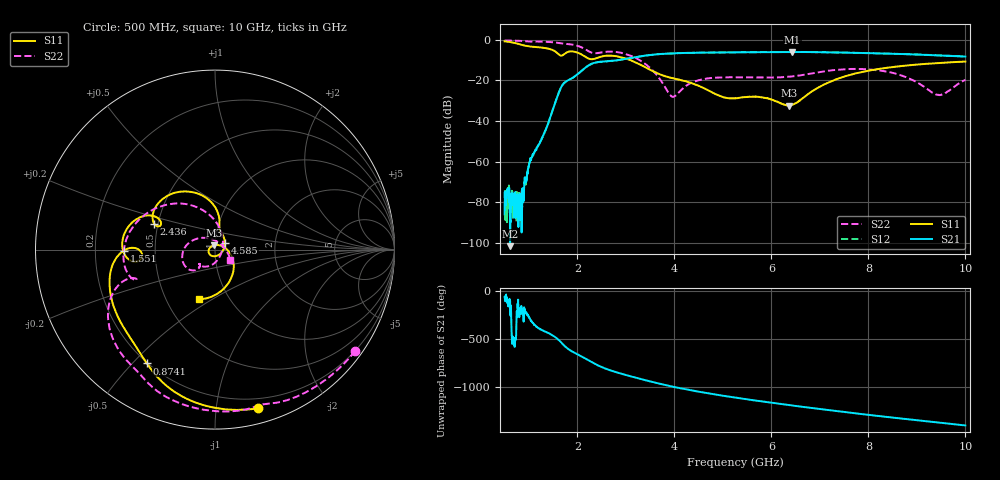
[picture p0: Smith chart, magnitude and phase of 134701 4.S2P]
!  2-Port S-parameters saved by WinCal
! VAR MeasName=S-Parameters (CALIBRATED_DATA) read from VNA (N5242A)
! VAR MeasDate=2013-7-3 16:21:27
! VAR NAME=134701 4
! VAR FILENAME=134701 4.S2P
! VAR DATE=2013-7-3 16:21:27
! VAR PHYS_PORTS=1,2
# Hz S MA R 50
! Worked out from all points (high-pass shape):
!   1601 points, 500 MHz to 10 GHz, reference 50 ohm
!   highest |S21| = -5.99 dB at 6.432 GHz (marker M1); lowest = -101.7 dB at 612.8 MHz (marker M2)
!   |S21| within 3 dB of the highest: 3.093 GHz to end of sweep
!   lowest |S11| = -32.5 dB at 6.372 GHz (marker M3), VSWR 1.05, Z = 49.4 + j2.27 ohm
!   |S11| at or under -10 dB: 3.09 GHz to end of sweep
!   |S22| runs from -28.1 to -0.3 dB; largest |S21 - S12| = 0.0033
!   S11 on the Smith chart (normalised r, x): 500 MHz: 0.12, -1.30; 874.1 MHz: 0.20, -0.55; 1.551 GHz: 0.33, -0.01; 2.436 GHz: 0.48, +0.16; 4.585 GHz: 1.11, +0.08; 10 GHz: 0.72, -0.44
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5e8  0.9167 -74.9  4.969e-05 -68.2  0.00013 -95.6  0.9631 -35.9
6.128125e8  0.8805 -90.3  8.261e-06 -99.5  0.0001217 127.1  0.9562 -43.9
8.146875e8  0.7737 -115.2  0.0001617 178.9  0.0001131 -93.5  0.9411 -58.3
8.740625e8  0.7392 -120.9  9.819e-05 133.8  0.0001366 -178.6  0.9336 -62.6
1.040312e9  0.6808 -134.0  0.0011 49.1  0.001188 45.1  0.902 -73.4
1.550938e9  0.5084 -179.3  0.03008 -124.7  0.03008 -125.0  0.8558 -111.1
1.717188e9  0.4327 -171.4  0.08399 155.2  0.08367 154.9  0.8031 -123.0
2.085312e9  0.4361 154.5  0.1719 36.8  0.1711 36.7  0.6527 -154.0
2.435625e9  0.3681 157.0  0.2838 -59.4  0.2828 -59.5  0.4743 -158.9
2.785938e9  0.3969 129.7  0.3098 -125.8  0.3089 -125.7  0.5042 177.2
3.118438e9  0.3065 102.6  0.3598 -173.5  0.3593 -173.3  0.3971 143.8
3.670625e9  0.1461 79.9  0.4431 115.2  0.4425 115.2  0.1206 77.1
3.973438e9  0.1129 76.0  0.4647 80.7  0.4646 80.8  0.0396 -17.4
4.585e9  0.06613 34.3  0.4826 21.7  0.4823 21.7  0.1066 -117.5
5.25e9  0.03643 -79.5  0.4917 -32.4  0.4919 -32.4  0.1195 -135.1
6.372188e9  0.02365 103.4  0.5005 -111.2  0.5011 -111.3  0.1234 -132.8
6.431562e9  0.02519 87.6  0.5016 -115.3  0.5009 -115.2  0.1253 -132.4
6.835312e9  0.05341 13.6  0.4979 -141.6  0.4975 -141.5  0.1488 -131.9
7.571562e9  0.1316 -37.8  0.4816 173.1  0.4816 173.1  0.1899 -150.9
8.420625e9  0.2072 -70.9  0.4559 123.6  0.4553 123.6  0.1613 171.5
9.441875e9  0.2686 -96.8  0.4129 66.8  0.4153 66.8  0.04414 57.4
1e10  0.2906 -108.3  0.3866 37.2  0.388 37.1  0.1038 -34.7
